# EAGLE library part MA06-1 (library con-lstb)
PIN HEADER
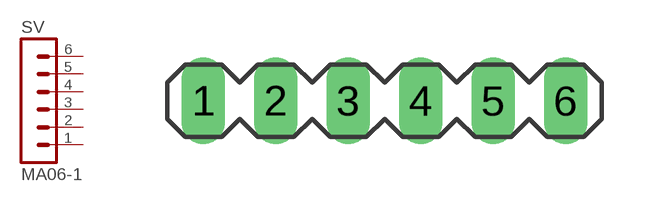
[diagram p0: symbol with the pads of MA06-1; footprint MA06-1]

Designator prefix SV

## MA06-1 (OC_FARNELL: unknown; OC_NEWARK: unknown)  [MA06-1]
1  1  pas
2  2  pas
3  3  pas
4  4  pas
5  5  pas
6  6  pas

## Footprint MA06-1 (pad centres in mm)
PIN HEADER
drill 1.016 long: 1 -6.35,0; 2 -3.81,0; 3 -1.27,0; 4 1.27,0; 5 3.81,0; 6 6.35,0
